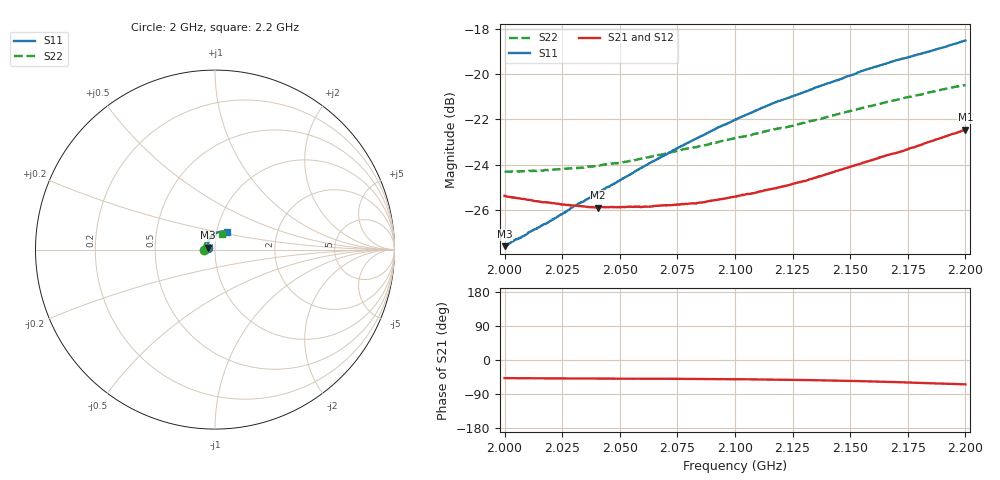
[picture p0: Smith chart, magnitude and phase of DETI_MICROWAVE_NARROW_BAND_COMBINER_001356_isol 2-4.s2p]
! 12/28/2020 4:18:56 PM
! \\DETI-AD\SERVEUR COMMUN\0\01 - PRODUIT\0 01 356 - COMBINEUR 4 VOIES BANDE S 800 WATTS\81 -PROCES VERBAL DE CONTROLE\MESURES\07 - S2P\ISOL 2-4.S2P
! CHANNEL.1
! TR.MEASUREMENT
! CORRECTED.DATA
# GHZ S RI R 50.0
! FREQ.GHZ  S11RE  S11IM  S21RE  S21IM  S12RE  S12IM  S22RE  S22IM
!; PortSelection: Port_12
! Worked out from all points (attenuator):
!   1000 points, 2 GHz to 2.2 GHz, reference 50 ohm
!   highest |S21| = -22.47 dB at 2.2 GHz (marker M1); lowest = -25.9 dB at 2.041 GHz (marker M2)
!   lowest |S11| = -27.6 dB at 2 GHz (marker M3), VSWR 1.09, Z = 46.1 + j1.03 ohm
!   |S11| at or under -10 dB: start of sweep to end of sweep
!   |S22| runs from -24.3 to -20.5 dB; largest |S21 - S12| = 0.00039
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2  -0.0402 0.0112  0.0362 -0.0399  0.0363 -0.04  -0.0607 -0.00417
2.013213  -0.0406 0.0204  0.0348 -0.0392  0.035 -0.0394  -0.0609 0.00529
2.018619  -0.0402 0.0242  0.0345 -0.039  0.0347 -0.0391  -0.0606 0.00924
2.024224  -0.04 0.0282  0.0341 -0.0387  0.0342 -0.0388  -0.0602 0.0132
2.03023  -0.0395 0.0324  0.0338 -0.0385  0.0338 -0.0387  -0.0595 0.0173
2.033433  -0.039 0.0345  0.0336 -0.0385  0.0337 -0.0386  -0.0589 0.0196
2.040641  -0.0378 0.0395  0.0332 -0.0383  0.0334 -0.0386  -0.0575 0.0251
2.052653  -0.035 0.0479  0.0331 -0.0386  0.0331 -0.0388  -0.0547 0.0333
2.059459  -0.0331 0.0526  0.0331 -0.0387  0.0331 -0.0388  -0.0527 0.038
2.066667  -0.0307 0.0574  0.0332 -0.0389  0.0333 -0.0389  -0.0505 0.0429
2.073473  -0.0282 0.0618  0.0333 -0.0392  0.0333 -0.0392  -0.048 0.0473
2.083083  -0.0241 0.0678  0.0333 -0.0397  0.0334 -0.04  -0.0439 0.053
2.091091  -0.0204 0.0726  0.0335 -0.0406  0.0336 -0.0407  -0.0403 0.0577
2.1001  -0.0155 0.0777  0.0339 -0.0415  0.034 -0.0417  -0.0355 0.0628
2.116717  -0.00564 0.0861  0.0347 -0.0437  0.0347 -0.0438  -0.0255 0.0709
2.123123  -0.00139 0.0885  0.0349 -0.0449  0.0348 -0.045  -0.0212 0.0734
2.133534  0.00621 0.0923  0.0352 -0.047  0.0351 -0.0471  -0.0138 0.0775
2.155155  0.0237 0.0987  0.0355 -0.0527  0.0356 -0.0526  0.00284 0.084
2.166767  0.0337 0.1003  0.0354 -0.0561  0.0352 -0.0561  0.0124 0.086
2.172172  0.0386 0.1008  0.035 -0.0577  0.0349 -0.0577  0.0171 0.0865
2.191391  0.0569 0.0996  0.0335 -0.0646  0.0337 -0.0646  0.0337 0.0863
2.2  0.0655 0.0988  0.0327 -0.0678  0.0328 -0.0679  0.0413 0.085
